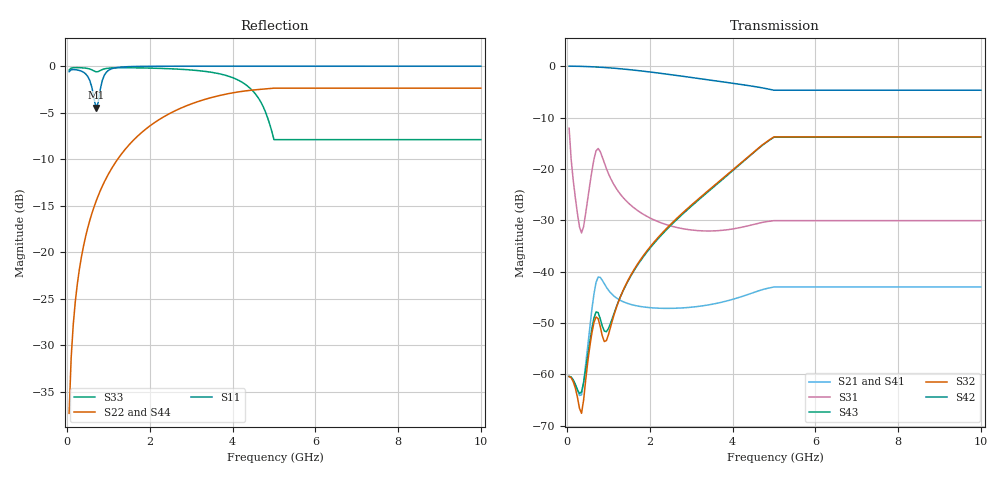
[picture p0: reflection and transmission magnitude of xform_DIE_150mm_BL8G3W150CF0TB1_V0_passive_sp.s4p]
! Created Wed Dec 13 16:24:39 2017
# ghz S ma R 50
! 4 Port Network Data from SP1.SP block
! freq  magS11  angS11  magS12  angS12  magS13  angS13  magS14  angS14
!  magS21  angS21  magS22  angS22  magS23  angS23  magS24  angS24
!  magS31  angS31  magS32  angS32  magS33  angS33  magS34  angS34
!  magS41  angS41  magS42  angS42  magS43  angS43  magS44  angS44
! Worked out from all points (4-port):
!   200 points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, 50 MHz to 10 GHz, reference 50 ohm
!   strongest paths, dB at 50 MHz, 2.55 GHz, 5.05 GHz, 7.55 GHz, 10 GHz:
!     S42: 0.0, -1.7, -4.7, -4.7, -4.7
!     S32: -60.5, -30.4, -13.8, -13.8, -13.8
!     S43: -60.4, -30.7, -13.8, -13.8, -13.8
!     S31: -12.1, -31.2, -30.1, -30.1, -30.1
!     S21: -60.5, -47.2, -43.0, -43.0, -43.0
!     S41: -60.5, -47.2, -43.1, -43.1, -43.1
!   lowest |S11| = -4.5 dB at 700 MHz (marker M1), VSWR 3.96, Z = 12.6 - j0.654 ohm
!   |S11| at or under -10 dB: nowhere
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0.05  0.9336 -165.8  0.0009448 18.0  0.2485 -72.8  0.0009402 18.0
      0.0009448 18.0  0.01365 90.8  0.0009479 17.8  0.9999 0.8
      0.2485 -72.8  0.0009479 17.8  0.9527 -165.5  0.0009552 19.9
      0.0009402 18.0  0.9999 0.8  0.0009552 19.9  0.01365 90.8
0.35  0.9389 177.4  0.0006297 76.2  0.02376 -19.3  0.0006266 76.2
      0.0006297 76.2  0.09513 95.4  0.0004161 83.4  0.9955 5.5
      0.02376 -19.3  0.0004161 83.4  0.9798 -179.8  0.0006722 85.9
      0.0006266 76.2  0.9955 5.5  0.0006722 85.9  0.09513 95.5
0.7  0.5969 -178.4  0.007819 93.3  0.1495 -7.4  0.00778 93.4
     0.007819 93.3  0.1876 100.8  0.00361 123.8  0.9821 10.8
     0.1495 -7.4  0.00361 123.8  0.9319 178.5  0.004033 119.7
     0.00778 93.4  0.9821 10.8  0.004033 119.7  0.1876 100.9
0.95  0.9273 -165.9  0.007046 35.1  0.1007 -69.4  0.00701 35.1
      0.007046 35.1  0.2509 104.5  0.002122 143.5  0.9679 14.5
      0.1007 -69.4  0.002122 143.5  0.9717 179.0  0.002592 131.0
      0.00701 35.1  0.9679 14.5  0.002592 131.0  0.2509 104.6
2.25  0.9984 -176.6  0.004388 28.0  0.03006 -93.4  0.004361 28.1
      0.004388 28.0  0.5203 121.3  0.02259 -161.2  0.853 31.3
      0.03006 -93.4  0.02259 -161.2  0.9724 171.4  0.02197 -165.1
      0.004361 28.1  0.853 31.3  0.02197 -165.1  0.5203 121.5
5  0.9989 -178.6  0.007076 -6.4  0.03129 -149.8  0.006996 -6.1
   0.007076 -6.4  0.7613 144.2  0.2048 168.0  0.583 49.2
   0.03129 -149.8  0.2048 168.0  0.4028 115.2  0.2033 167.3
   0.006996 -6.1  0.583 49.2  0.2033 167.3  0.7623 144.5
10  0.9989 -178.6  0.007076 -6.4  0.03129 -149.8  0.006996 -6.1
    0.007076 -6.4  0.7613 144.2  0.2048 168.0  0.583 49.2
    0.03129 -149.8  0.2048 168.0  0.4028 115.2  0.2033 167.3
    0.006996 -6.1  0.583 49.2  0.2033 167.3  0.7623 144.5
